PROGRAM MAIN

VAR CONSTANT	
	cInitSource			: ST_MA_MultiArray_InitPars 
							:= (eTypeCode := eMA_TypeCode_LREAL, nDims := 2, aDimSizes := [cChannels, cBufferLength]);	
END_VAR

VAR
	fbErrHist		: FB_HRErrHist; 					// error monitoring	
	
	fbNoiseGeneratorCh1		: FB_NoiseGenerator;		// Signal Generator
	fbNoiseGeneratorCh2		: FB_NoiseGenerator;		// Signal Generator	
	fbFunctionGeneratorCh3	: FB_FunctionGenerator;		// Signal Generator	
	
	aBuffer			: ARRAY[1..cChannels] OF ARRAY[1..cOversamples] OF LREAL;
	
	nStartSeed		: INT := 1;	
	aNormDisp		: ARRAY [1..2] OF LREAL := [1,3];	// mean = 1, std = 3
	aGammaDisp      : ARRAY [1..2] OF LREAL := [4,0];   // DOF = 4
	fSetFrequency	: LREAL := 40;						// Hz
	fSetAmplitude	: LREAL := 10;						// peak amplitude of sine signal	
	
	fbSource 		: FB_CMA_Source := (stInitPars 	:= cInitSource, 
										nOwnID 		:= eID_Source, 
										aDestIDs 	:= [eID_Histogram, eID_Mean, eID_Std, eID_Skew, eID_ExcessKurtosis],
										nResultBuffers := 8);
END_VAR

// Generate test signals
// Ch1: Normal distribution
// Ch2: Gamma distribution
// Ch3: Sine signal
fbNoiseGeneratorCh1(	nSeed 		:= nStartSeed,
						aParam 		:= aNormDisp,
						eDistrType	:= E_DistributionType.Normal,								
						aSignal		:= aBuffer[1] );	
fbNoiseGeneratorCh2(	nSeed 		:= nStartSeed,
						aParam 		:= aGammaDisp,
						eDistrType	:= E_DistributionType.Gamma,								
						aSignal		:= aBuffer[2] );									
fbFunctionGeneratorCh3(	fFrequency 	:= fSetFrequency,
						fAmplitude 	:= fSetAmplitude,
						fOffset		:= 0,
						eFunction 	:= E_FunctionType.Sine,							
						aSignal		:= aBuffer[3] );	

// Call source to collect data
fbSource.Input2D( pDataIn 			:= ADR(aBuffer),
				  nDataInSize 		:= SIZEOF(aBuffer), 
				  eElementType 		:= eMA_TypeCode_LREAL,
				  nWorkDim0			:= 0,
				  nWorkDim1 		:= 1,				  				  
				  pStartIndex		:= 0,
				  nOptionPars		:= 0 );	  
IF fbSource.bError THEN
	fbErrHist.AddError(bErr := TRUE, hrErrCode := fbSource.hrErrorCode, sErrSource := 'MAIN.fbSource'); 
	// ToDo: if error
END_IF

END_PROGRAM
